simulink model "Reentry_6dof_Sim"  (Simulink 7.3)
settings: Solver=ode45  StartTime=0.0  StopTime=1943  FixedStep=0.01
InitFcn:
  | init
StopFcn:
  | pl
  | save_traj
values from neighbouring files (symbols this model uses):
  d2r = pi/180    (= 0.0174532925199)    [init.m]    (also in pl.m; robust.m)
  h0 = 250000.0    (= 250000)    [init.m]
  mass = 528.0    (= 528)    [init.m]
  r2d = 180/pi    (= 57.2957795131)    [init.m]    (also in pl.m; robust.m)
  sp = 15    [init.m]
  x0 = [0 0 -2 -2 0 0 18 0 0 0]'*d2r    [init.m]
  x_cg = -17.04    [init.m]
  x_ref = -16.2    [init.m]
  y_cg = 0    [init.m]
  z_cg = -2.03    [init.m]
  z_ref = -2.1    [init.m]
undefined symbols (not defined in the file or in its folder): Cl, Cld1, Cld2, Cld3, Cld4, Cld5, Cld6, Cld7, Cm, Cmd1, Cmd2, Cmd3, Cmd4, Cmd5, Cmd6, Cmd7, Cn, Cnd1, Cnd2, Cnd3, Cnd4, Cnd5, Cnd6, Cnd7, CX, CXd1, CXd2, CXd3, CXd4, CXd5, CXd6, CXd7, CY, CYd1, CYd2, CYd3, CYd4, CYd5, CYd6, CYd7, CZ, CZd1, CZd2, CZd3, CZd4, CZd5, CZd6, CZd7, ft, HDBK, km, Lateral_FCS, MIL, Pitch_FCS, sigbuilder_block
libraries: aerolibasang x3, aerolib6dof2 x1, aerolibconvert2 x1, aerolibatmos2 x1, aerolibgravity2 x1, aerolibadyn x1
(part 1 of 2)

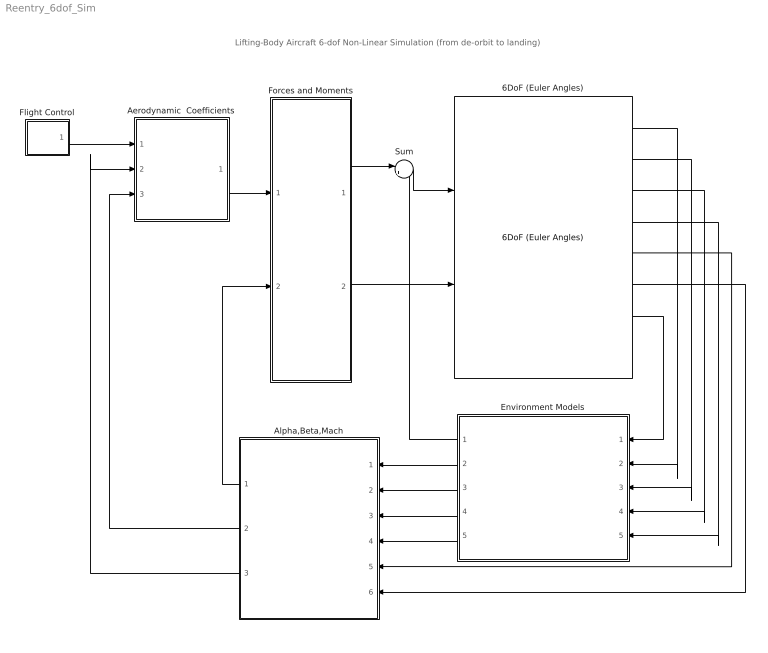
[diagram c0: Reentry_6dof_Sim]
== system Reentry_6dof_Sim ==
  note: Lifting-Body Aircraft 6-dof Non-Linear Simulation (from de-orbit to landing)
  6DoF (Euler Angles) : aerolib6dof2/6DoF (Euler Angles)  SystemSampleTime=-1  units=English (Velocity in ft/s)  mtype=Fixed  rep=Euler Angles  xme_0=[-x0, 0, -h0]  Vm_0=Uvw_0  eul_0=Euler_0  pm_0=pqr_0  mass_0=mass  mass_e=0.5  mass_f=2.0  inertia=inertia  inertia_e=eye(3)  inertia_f=2*eye(3)  k_quat=1.0
  Aerodynamic  Coefficients : Subsystem
  Alpha,Beta,Mach : Subsystem
  Environment Models : Subsystem
  Flight Control : Subsystem
  Forces and Moments : Subsystem
  Sum : Sum  Inputs=|++  OutDataType=sfix(16)  OutScaling=2^0
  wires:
  6DoF (Euler Angles)/5 -> Alpha,Beta,Mach/5(Vb)
  6DoF (Euler Angles)/1 -> Environment Models/2(Ve)
  6DoF (Euler Angles)/2 -> Environment Models/3(Xe)
  6DoF (Euler Angles)/3 -> Environment Models/4(Euler)
  6DoF (Euler Angles)/4 -> Environment Models/5(DCM)
  Sum/1 -> 6DoF (Euler Angles)/1
  Forces and Moments/1(X,Y,Z) -> Sum/1
  Environment Models/2(Speed of Sound) -> Alpha,Beta,Mach/1(Speed of Sound)
  Environment Models/3(Wind Velocity) -> Alpha,Beta,Mach/2(Wind Velocity)
  Environment Models/4(Air Density) -> Alpha,Beta,Mach/3(Air Density)
  Environment Models/5(Wind Angular Rates) -> Alpha,Beta,Mach/4(Wind Angular Rates)
  6DoF (Euler Angles)/6 -> Alpha,Beta,Mach/6(p,q,r)
  Forces and Moments/2(LMN) -> 6DoF (Euler Angles)/2
  6DoF (Euler Angles)/7 -> Environment Models/1(omgd)
  Environment Models/1(Fg) -> Sum/2
  Alpha,Beta,Mach/1(qbar) -> Forces and Moments/2(qbar)
  Aerodynamic  Coefficients/1(Coeff) -> Forces and Moments/1(Coeff)
  Alpha,Beta,Mach/2(Mach) -> Aerodynamic  Coefficients/3(Mach)
  Alpha,Beta,Mach/3(Incid) -> Aerodynamic  Coefficients/2(Incid)
  Flight Control/1(delta) -> Aerodynamic  Coefficients/1(deltas)

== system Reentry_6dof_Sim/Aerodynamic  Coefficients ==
  note: Aero Coefficients, funct. of: (Alpha, Beta, Mach#, Deflection)
  deltas : Inport  OutDataType=sfix(16)  OutScaling=2^0
  Incid : Inport  Port=2  OutDataType=sfix(16)  OutScaling=2^0
  Mach : Inport  Port=3  OutDataType=sfix(16)  OutScaling=2^0
  Aero-Surface Coefficient Increments : Subsystem
  Angle Conversion : aerolibconvert2/Angle Conversion  SystemSampleTime=-1  IU=rad  OU=deg
  Base Aero  Coefficients : Subsystem
  Sum : Sum  Inputs=|++  OutDataType=fixdt(1, 16)  OutScaling=2^0
  albet : Scope
  delta : Scope
  Coeff : Outport  OutDataType=sfix(16)  OutScaling=2^0  InitialOutput=0
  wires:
  deltas/1 -> Aero-Surface Coefficient Increments/3(delta), delta/1
  Base Aero  Coefficients/1(Coeff) -> Sum/1
  Sum/1 -> Coeff/1
  Mach/1 -> Base Aero  Coefficients/2(Mach), Aero-Surface Coefficient Increments/2(Mach)
  Angle Conversion/1 -> Base Aero  Coefficients/1(albet), albet/1, Aero-Surface Coefficient Increments/1(albet)
  Incid/1 -> Angle Conversion/1
  Aero-Surface Coefficient Increments/1(Coeff) -> Sum/2

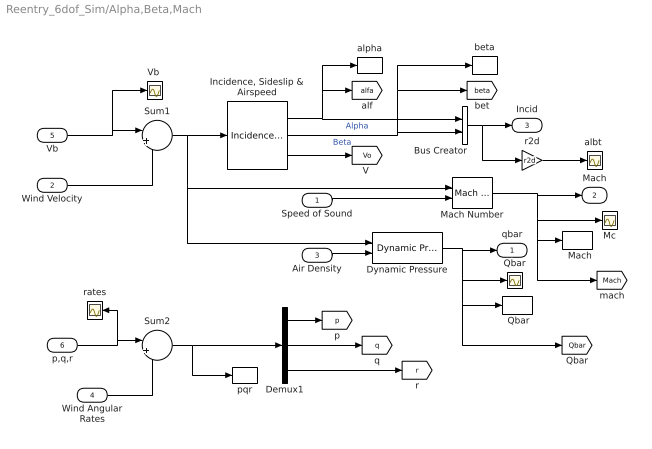
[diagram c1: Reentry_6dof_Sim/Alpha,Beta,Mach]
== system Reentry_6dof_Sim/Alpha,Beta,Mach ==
  Speed of Sound : Inport  OutDataType=sfix(16)  OutScaling=2^0
  Wind Velocity : Inport  Port=2  PortDimensions=3  OutDataType=sfix(16)  OutScaling=2^0
  Air Density : Inport  Port=3  OutDataType=sfix(16)  OutScaling=2^0
  Wind Angular Rates : Inport  Port=4  PortDimensions=3  OutDataType=sfix(16)  OutScaling=2^0
  Vb : Inport  Port=5  PortDimensions=3  OutDataType=sfix(16)  OutScaling=2^0
  p,q,r : Inport  Port=6  PortDimensions=3  OutDataType=sfix(16)  OutScaling=2^0
  "  Mach" : ToWorkspace  VariableName=Mach  SampleTime=-1  SaveFormat=Array
  " Qbar" : ToWorkspace  VariableName=Qbar  SampleTime=-1  SaveFormat=Array
  Bus Creator : BusCreator  Inputs=2
  Demux1 : Demux  Outputs=3
  Dynamic Pressure : aerolibasang/Dynamic Pressure  SystemSampleTime=-1
  "Incidence, Sideslip & Airspeed" : aerolibasang/Incidence, Sideslip, & Airspeed  SystemSampleTime=-1
  Mach Number : aerolibasang/Mach Number  SystemSampleTime=-1
  Mc : Scope
  Qbar : Scope
  Sum1 : Sum  Inputs=|+-  OutDataType=sfix(16)  OutScaling=2^0
  Sum2 : Sum  Inputs=|++  OutDataType=sfix(16)  OutScaling=2^0
  "Vb " : Scope
  "albt " : Scope
  alpha : ToWorkspace  VariableName=alfa  SampleTime=-1  SaveFormat=Array
  beta : ToWorkspace  VariableName=beta  SampleTime=-1  SaveFormat=Array
  pqr : ToWorkspace  VariableName=pqr  SampleTime=-1  SaveFormat=Array
  r2d : Gain  Gain=r2d  ParameterDataType=sfix(16)  ParameterScaling=2^0  OutDataType=sfix(16)  OutScaling=2^0
  rates : Scope
  qbar : Outport  OutDataType=sfix(16)  OutScaling=2^0  InitialOutput=0
  Mach : Outport  Port=2  OutDataType=sfix(16)  OutScaling=2^0
  Incid : Outport  Port=3  OutDataType=sfix(16)  OutScaling=2^0
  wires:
  Demux1/1 -> [p]
  Demux1/3 -> [r]
  Demux1/2 -> [q]
  Sum2/1 -> pqr/1, Demux1/1
  Wind Angular Rates/1 -> Sum2/2
  p,q,r/1 -> rates/1, Sum2/1
  "Incidence, Sideslip & Airspeed"/1 -> alpha/1, [alfa], Bus Creator/1  "Alpha"
  Bus Creator/1 -> Incid/1, r2d/1
  "Incidence, Sideslip & Airspeed"/2 -> beta/1, [beta], Bus Creator/2  "Beta"
  Wind Velocity/1 -> Sum1/2
  Speed of Sound/1 -> Mach Number/2
  Vb/1 -> "Vb "/1, Sum1/1
  Sum1/1 -> "Incidence, Sideslip & Airspeed"/1, Mach Number/1, Dynamic Pressure/1
  Mach Number/1 -> [Mach], "  Mach"/1, Mc/1, Mach/1
  Air Density/1 -> Dynamic Pressure/2
  Dynamic Pressure/1 -> [Qbar], " Qbar"/1, Qbar/1, qbar/1
  "Incidence, Sideslip & Airspeed"/3 -> [Vo]
  r2d/1 -> "albt "/1

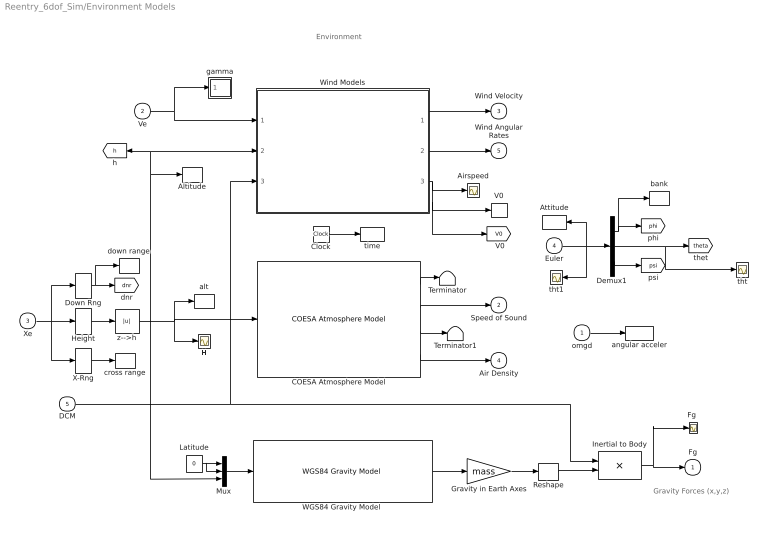
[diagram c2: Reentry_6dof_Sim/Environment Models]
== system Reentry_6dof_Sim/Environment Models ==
  note: Gravity Forces (x,y,z)
  note: Environment
  omgd : Inport  OutDataType=sfix(16)  OutScaling=2^0
  Ve : Inport  Port=2  OutDataType=sfix(16)  OutScaling=2^0
  Xe : Inport  Port=3  PortDimensions=3  OutDataType=sfix(16)  OutScaling=2^0
  Euler : Inport  Port=4  OutDataType=sfix(16)  OutScaling=2^0
  DCM : Inport  Port=5  OutDataType=sfix(16)  OutScaling=2^0
  Airspeed : Scope
  Altitude : ToWorkspace  VariableName=Alt  SampleTime=-1  SaveFormat=Array
  Attitude : ToWorkspace  VariableName=Euler  SampleTime=-1  SaveFormat=Array
  COESA Atmosphere Model : aerolibatmos2/COESA Atmosphere Model  SystemSampleTime=-1  units=English (Velocity in ft/s)  spec=MIL-HDBK-310  model=Profile  profile_var=High temperature  profile_percent=1%  profile_alt=40 km (131234 ft)  envelope_var=High temperature  envelope_percent=1%  action=Warning
  Clock : Clock
  Demux1 : Demux  Outputs=3
  Down Rng : Selector  InputPortWidth=3  IndexOptions=Index vector (dialog)  Indices=[1]  OutputSizes=1
  "Fg " : Scope
  Gravity in Earth Axes : Gain  Gain=mass  ParameterDataType=sfix(16)  ParameterScaling=2^0  OutDataType=sfix(16)  OutScaling=2^0
  H : Scope
  Height : Selector  InputPortWidth=3  IndexOptions=Index vector (dialog)  Indices=[3]  OutputSizes=1
  Inertial to Body : Product  Multiplication=Matrix(*)  OutDataType=sfix(16)  OutScaling=2^0
  Latitude : Constant  Value=0  OutDataType=sfix(16)  OutScaling=2^0
  Mux : Mux  Inputs=3
  Reshape : Reshape
  Terminator : Terminator
  Terminator1 : Terminator
  V0 : ToWorkspace  VariableName=V0  SampleTime=-1  SaveFormat=Array
  "WGS84 Gravity Model " : aerolibgravity2/WGS84 Gravity Model   SystemSampleTime=-1  model=WGS84 Taylor Series  units=English  no_atmos=on  precessing=on  jd_loc=off  month=October  day=10  year=2004  no_centrifugal=on  action=None
  Wind Models : Subsystem
  X-Rng : Selector  InputPortWidth=3  IndexOptions=Index vector (dialog)  Indices=[2]  OutputSizes=1
  alt : ToWorkspace  VariableName=alt  SampleTime=-1  SaveFormat=Array
  angular acceler : ToWorkspace  VariableName=omgd  SampleTime=-1  SaveFormat=Array
  bank : ToWorkspace  VariableName=phi  SampleTime=-1  SaveFormat=Array
  cross range : ToWorkspace  VariableName=xrng  SampleTime=-1  SaveFormat=Array
  down range : ToWorkspace  VariableName=dnr  SampleTime=-1  SaveFormat=Array
  gamma : Subsystem
  tht : Scope
  tht1 : Scope
  time : ToWorkspace  VariableName=time  SampleTime=-1  SaveFormat=Array
  z-->h : Abs
  Fg : Outport  OutDataType=sfix(16)  OutScaling=2^0  InitialOutput=0
  Speed of Sound : Outport  Port=2  OutDataType=sfix(16)  OutScaling=2^0  InitialOutput=0
  Wind Velocity : Outport  Port=3  OutDataType=sfix(16)  OutScaling=2^0  InitialOutput=0
  Air Density : Outport  Port=4  OutDataType=sfix(16)  OutScaling=2^0  InitialOutput=0
  Wind Angular Rates : Outport  Port=5  OutDataType=sfix(16)  OutScaling=2^0  InitialOutput=0
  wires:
  Reshape/1 -> Inertial to Body/2
  "WGS84 Gravity Model "/1 -> Gravity in Earth Axes/1
  Gravity in Earth Axes/1 -> Reshape/1
  COESA Atmosphere Model/1 -> Terminator/1
  COESA Atmosphere Model/2 -> Speed of Sound/1
  COESA Atmosphere Model/3 -> Terminator1/1
  COESA Atmosphere Model/4 -> Air Density/1
  DCM/1 -> Inertial to Body/1, Wind Models/3(DCM)
  Inertial to Body/1 -> Fg/1, "Fg "/1
  Mux/1 -> "WGS84 Gravity Model "/1
  Latitude/1 -> Mux/2, Mux/1
  Height/1 -> z-->h/1
  Xe/1 -> Height/1, Down Rng/1, X-Rng/1
  z-->h/1 -> COESA Atmosphere Model/1, H/1, alt/1, Mux/3, Wind Models/2(Altitude), [h], Altitude/1
  Wind Models/2(pg,qg,rg) -> Wind Angular Rates/1
  Wind Models/3(Airspeed) -> Airspeed/1, V0/1, [V0]
  Ve/1 -> Wind Models/1(Ve), gamma/1(Ve)
  Wind Models/1(ug,vg,wg) -> Wind Velocity/1
  Down Rng/1 -> [dnr], down range/1
  Clock/1 -> time/1
  X-Rng/1 -> cross range/1
  omgd/1 -> angular acceler/1
  Euler/1 -> Demux1/1, Attitude/1, tht1/1
  Demux1/2 -> [theta], tht/1
  Demux1/1 -> [phi], bank/1
  Demux1/3 -> [psi]

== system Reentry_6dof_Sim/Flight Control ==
  note: Surface Open-Loop Trim Commands and Closed-Loop Flight Control
  Bus Creator2 : BusCreator  Inputs=7
  Deflection Limits : Subsystem
  Demux1 : Demux  Outputs=7
  Flight  Control : Subsystem
  Sum1 : Sum  Inputs=|++  OutDataType=fixdt(1, 16)  OutScaling=2^0
  Trim Cmds : Subsystem
  delta : Outport
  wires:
  Trim Cmds/1(Trim) -> Sum1/2
  Flight  Control/1(deltas) -> Sum1/1
  Sum1/1 -> Deflection Limits/1(In)
  Demux1/1 -> Bus Creator2/1  "Left_Elevon"
  Bus Creator2/1 -> delta/1
  Demux1/2 -> Bus Creator2/2  "Right_Elevon"
  Demux1/3 -> Bus Creator2/3  "Vert_Rudder"
  Demux1/6 -> Bus Creator2/6  "Bflap_LoLft"
  Demux1/7 -> Bus Creator2/7  "Bflap_LoRht"
  Demux1/5 -> Bus Creator2/5  "Bflap_UpRht"
  Demux1/4 -> Bus Creator2/4  "Bflap_UpLft"
  Deflection Limits/1(Ou) -> Demux1/1

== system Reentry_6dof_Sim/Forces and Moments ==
  note: Aero coefficients (CX,CY,CZ,Cl,Cm,Cn)
  note: Dynamic Pressure
  note: Moments and Forces due to Aero and Engine Thrust
  Coeff : Inport  OutDataType=sfix(16)  OutScaling=2^0
  qbar : Inport  Port=2  OutDataType=sfix(16)  OutScaling=2^0
  Acceler X,Y,Z : Scope
  Aero-Forcces : Selector  InputPortWidth=3  IndexOptions=Index vector (dialog)  Indices=[3,1,2]  OutputSizes=1
  "Aerodynamic Forces and Moments (Fx,Fy,Fz), (Lx,My,Nz)" : aerolibadyn/Aerodynamic Forces and Moments   SystemSampleTime=-1  inputAxes=Body  outputForceAxes=Body  outputMomentAxes=Body  S=Sref  b=sp  cbar=ch
  Axyz : ToWorkspace  VariableName=Axyz  SampleTime=-1  SaveFormat=Array
  "Center of Gravity plus Variation [x_cg, y_cg,  z_cg]" : Step  Time=0  Before="[x_cg, y_cg,  z_cg]"  After="[x_cg,   y_cg,   z_cg]"
  Faero : ToWorkspace  VariableName=Flds  SampleTime=-1  SaveFormat=Array
  "Force " : Scope
  Force ---> Acc : Gain  Gain=1/mass  ParameterDataType=sfix(16)  ParameterScaling=2^0  OutDataType=sfix(16)  OutScaling=2^0
  Moments : Scope
  Moments Reference Center (MRC) in (feet) : Constant  Value=[x_ref 0 z_ref]  OutDataType=sfix(16)  OutScaling=2^0
  Nz : Selector  InputPortWidth=3  IndexOptions=Index vector (dialog)  Indices=[3]  OutputSizes=1
  X,Y,Z : Outport  OutDataType=sfix(16)  OutScaling=2^0  InitialOutput=0
  LMN : Outport  Port=2  OutDataType=sfix(16)  OutScaling=2^0  InitialOutput=0
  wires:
  Coeff/1 -> "Aerodynamic Forces and Moments (Fx,Fy,Fz), (Lx,My,Nz)"/1
  qbar/1 -> "Aerodynamic Forces and Moments (Fx,Fy,Fz), (Lx,My,Nz)"/2
  Moments Reference Center (MRC) in (feet)/1 -> "Aerodynamic Forces and Moments (Fx,Fy,Fz), (Lx,My,Nz)"/4
  "Center of Gravity plus Variation [x_cg, y_cg,  z_cg]"/1 -> "Aerodynamic Forces and Moments (Fx,Fy,Fz), (Lx,My,Nz)"/3
  Force ---> Acc/1 -> Acceler X,Y,Z/1, Axyz/1, Nz/1
  Aero-Forcces/1 -> Faero/1
  "Aerodynamic Forces and Moments (Fx,Fy,Fz), (Lx,My,Nz)"/2 -> LMN/1, Moments/1
  "Aerodynamic Forces and Moments (Fx,Fy,Fz), (Lx,My,Nz)"/1 -> Aero-Forcces/1, Force ---> Acc/1, X,Y,Z/1, "Force "/1
  Nz/1 -> [Nz]

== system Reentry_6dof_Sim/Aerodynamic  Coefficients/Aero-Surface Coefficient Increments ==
  note: Surface Coefficients
  albet : Inport
  Mach : Inport  Port=2
  delta : Inport  Port=3
  LL Bflap : Subsystem
  LR Bflap : Subsystem
  Left Elevon : Subsystem
  Right Elevon : Subsystem
  Rudder : Subsystem
  Sum : Sum  Inputs=+++++++  OutDataType=fixdt(1, 16)  OutScaling=2^0
  UL Bflap : Subsystem
  UR Bflap : Subsystem
  Coeff : Outport
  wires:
  Left Elevon/1(Coeff) -> Sum/1
  delta/1 -> Left Elevon/3(delta), Right Elevon/3(delta), Rudder/3(delta), UL Bflap/3(delta), UR Bflap/3(delta), LL Bflap/3(delta), LR Bflap/3(delta)
  albet/1 -> Left Elevon/1(albet), Right Elevon/1(albet), Rudder/1(albet), UL Bflap/1(albet), UR Bflap/1(albet), LL Bflap/1(albet), LR Bflap/1(albet)
  Mach/1 -> Left Elevon/2(Mach), Right Elevon/2(Mach), Rudder/2(Mach), UL Bflap/2(Mach), UR Bflap/2(Mach), LL Bflap/2(Mach), LR Bflap/2(Mach)
  Sum/1 -> Coeff/1
  Right Elevon/1(Coeff) -> Sum/2
  Rudder/1(Coeff) -> Sum/3
  UL Bflap/1(Coeff) -> Sum/4
  UR Bflap/1(Coeff) -> Sum/5
  LL Bflap/1(Coeff) -> Sum/6
  LR Bflap/1(Coeff) -> Sum/7

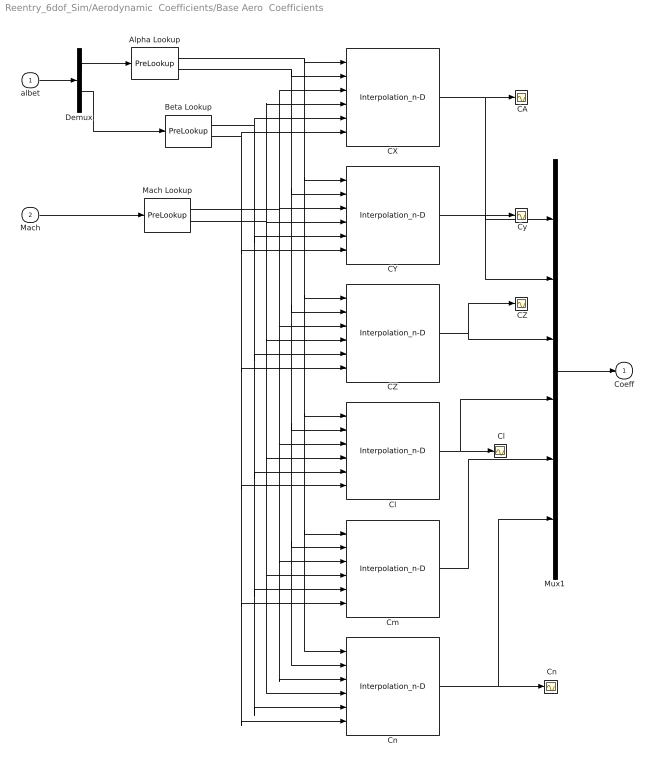
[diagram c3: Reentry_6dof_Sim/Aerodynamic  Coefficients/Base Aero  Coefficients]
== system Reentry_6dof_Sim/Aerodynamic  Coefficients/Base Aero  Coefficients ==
  albet : Inport  OutDataType=sfix(16)  OutScaling=2^0
  Mach : Inport  Port=2  OutDataType=sfix(16)  OutScaling=2^0
  " CA" : Scope
  " CZ" : Scope
  " Cl" : Scope
  " Cn" : Scope
  " Cy" : Scope
  Alpha Lookup : PreLookup  BreakpointsData=Alfas  BeginIndexSearchUsingPreviousIndexResult=on  ProcessOutOfRangeInput=Linear extrapolation  IndexDataType=sfix(16)  FractionDataType=sfix(16)  FractionScaling=2^0
  Beta Lookup : PreLookup  BreakpointsData=Betas  BeginIndexSearchUsingPreviousIndexResult=on  ProcessOutOfRangeInput=Linear extrapolation  IndexDataType=sfix(16)  FractionDataType=sfix(16)  FractionScaling=2^0
  CX : Interpolation_n-D  NumberOfTableDimensions=3  Table=CX  CheckIndexInCode=off  OutDataType=sfix(16)  OutScaling=2^0
  CY : Interpolation_n-D  NumberOfTableDimensions=3  Table=CY  CheckIndexInCode=off  OutDataType=sfix(16)  OutScaling=2^0
  CZ : Interpolation_n-D  NumberOfTableDimensions=3  Table=CZ  CheckIndexInCode=off  OutDataType=sfix(16)  OutScaling=2^0
  Cl : Interpolation_n-D  NumberOfTableDimensions=3  Table=Cl  CheckIndexInCode=off  OutDataTypeMode=double  OutDataType=sfix(16)  OutScaling=2^0  OutDataTypeStr=double
  Cm : Interpolation_n-D  NumberOfTableDimensions=3  Table=Cm  CheckIndexInCode=off  OutDataType=sfix(16)  OutScaling=2^0
  Cn : Interpolation_n-D  NumberOfTableDimensions=3  Table=Cn  CheckIndexInCode=off  OutDataType=sfix(16)  OutScaling=2^0
  Demux : Demux  Outputs=2
  Mach Lookup : PreLookup  BreakpointsData=Machs  BeginIndexSearchUsingPreviousIndexResult=on  ProcessOutOfRangeInput=Linear extrapolation  IndexDataType=sfix(16)  FractionDataType=sfix(16)  FractionScaling=2^0
  Mux1 : Mux  Inputs=6
  Coeff : Outport  OutDataType=sfix(16)  OutScaling=2^0  InitialOutput=0
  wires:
  Mach/1 -> Mach Lookup/1
  albet/1 -> Demux/1
  Demux/2 -> Beta Lookup/1
  Mux1/1 -> Coeff/1
  Beta Lookup/2 -> CZ/6, Cl/6, Cn/6, Cm/6, CY/6, CX/6
  Beta Lookup/1 -> CY/5, CZ/5, Cl/5, Cn/5, Cm/5, CX/5
  Mach Lookup/2 -> CX/4, CZ/4, Cl/4, Cn/4, Cm/4, CY/4
  Mach Lookup/1 -> CX/3, CZ/3, Cl/3, Cn/3, Cm/3, CY/3
  Alpha Lookup/2 -> Cn/2, Cm/2, Cl/2, CZ/2, CY/2, CX/2
  Alpha Lookup/1 -> CZ/1, Cl/1, Cn/1, Cm/1, CY/1, CX/1
  Cn/1 -> " Cn"/1, Mux1/6
  Cm/1 -> Mux1/5
  Cl/1 -> " Cl"/1, Mux1/4
  CZ/1 -> " CZ"/1, Mux1/3
  CY/1 -> " Cy"/1, Mux1/2
  CX/1 -> " CA"/1, Mux1/1
  Demux/1 -> Alpha Lookup/1

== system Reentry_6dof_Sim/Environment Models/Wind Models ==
  note: Wind Disturbance Model (Shear, Gust, Turbulence)
  Ve : Inport  OutDataType=sfix(16)  OutScaling=2^0
  Altitude : Inport  Port=2  OutDataType=sfix(16)  OutScaling=2^0
  DCM : Inport  Port=3  OutDataType=sfix(16)  OutScaling=2^0
  Dot Product : DotProduct  OutDataType=sfix(16)  OutScaling=2^-10  SaturateOnIntegerOverflow=on
  V : Math  Operator=sqrt  OutDataType=sfix(16)  OutScaling=2^0
  ug,vg,wg : Outport  OutDataType=sfix(16)  OutScaling=2^0
  pg,qg,rg : Outport  Port=2  OutDataType=sfix(16)  OutScaling=2^0
  Airspeed : Outport  Port=3  OutDataType=sfix(16)  OutScaling=2^0
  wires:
  Altitude/1 -> ?
  Dot Product/1 -> V/1
  Ve/1 -> Dot Product/1, Dot Product/2
  V/1 -> Airspeed/1

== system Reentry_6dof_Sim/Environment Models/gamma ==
  Ve : Inport
  -1 : Gain  Gain=-1  ParameterDataType=sfix(16)  ParameterScaling=2^0  OutDataType=sfix(16)  OutScaling=2^0
  57.2 : Gain  Gain=r2d  ParameterDataType=sfix(16)  ParameterScaling=2^0  OutDataType=sfix(16)  OutScaling=2^0
  Vx : Selector  InputPortWidth=3  IndexOptions=Index vector (dialog)  Indices=[1]  OutputSizes=1
  Vz : Selector  InputPortWidth=3  IndexOptions=Index vector (dialog)  Indices=[3]  OutputSizes=1
  atan : Trigonometry  Operator=atan2
  "gam " : Scope
  gama : ToWorkspace  VariableName=gama  SampleTime=-1  SaveFormat=Array
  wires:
  Vz/1 -> atan/1
  Vx/1 -> atan/2
  atan/1 -> 57.2/1
  57.2/1 -> "gam "/1, gama/1, [gama]
  -1/1 -> Vz/1
  Ve/1 -> -1/1, Vx/1

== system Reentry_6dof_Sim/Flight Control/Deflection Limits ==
  In : Inport
  "  Delta  (deg)" : ToWorkspace  VariableName=delta  SampleTime=-1  SaveFormat=Array
  Demux : Demux  Outputs=7
  LL BFlap : Saturate  UpperLimit=60  LowerLimit=0  OutDataType=fixdt(1, 16)  OutScaling=2^0
  LR BFlap : Saturate  UpperLimit=60  LowerLimit=0  OutDataType=fixdt(1, 16)  OutScaling=2^0
  Left Elev : Saturate  UpperLimit=30  LowerLimit=-30  OutDataType=fixdt(1, 16)  OutScaling=2^0
  Mux1 : Mux  Inputs=7
  Right Elev : Saturate  UpperLimit=30  LowerLimit=-30  OutDataType=fixdt(1, 16)  OutScaling=2^0
  UL BFlap : Saturate  UpperLimit=0  LowerLimit=-60  OutDataType=fixdt(1, 16)  OutScaling=2^0
  UR BFlap : Saturate  UpperLimit=0  LowerLimit=-60  OutDataType=fixdt(1, 16)  OutScaling=2^0
  Vert Rudder : Saturate  UpperLimit=40  LowerLimit=-40  OutDataType=fixdt(1, 16)  OutScaling=2^0
  Ou : Outport
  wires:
  Mux1/1 -> Ou/1, "  Delta  (deg)"/1
  In/1 -> Demux/1
  Demux/7 -> LR BFlap/1
  Demux/6 -> LL BFlap/1
  Demux/5 -> UR BFlap/1
  Demux/4 -> UL BFlap/1
  Demux/3 -> Vert Rudder/1
  Demux/2 -> Right Elev/1
  Demux/1 -> Left Elev/1
  LL BFlap/1 -> Mux1/6
  UR BFlap/1 -> Mux1/5
  UL BFlap/1 -> Mux1/4
  Vert Rudder/1 -> Mux1/3
  Right Elev/1 -> Mux1/2
  Left Elev/1 -> Mux1/1
  LR BFlap/1 -> Mux1/7

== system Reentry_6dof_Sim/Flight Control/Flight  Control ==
  note: Guidance Commands and Flight Control System
  note: 7 Aero-Surface Deflections
  Guidance Commands 1876 sec : Subsystem  Tag=STV Subsys  LoadFcn=sigbuilder_block('load');  StartFcn=sigbuilder_block('start');  StopFcn=sigbuilder_block('stop');  ClipboardFcn=sigbuilder_block('clipboard');
  Lateral Flight Control : Subsystem
  Pitch Flight Control : Subsystem
  Sum : Sum  Inputs=|+-  OutDataType=fixdt(1, 16)  OutScaling=2^0
  Sum1 : Sum  Inputs=|-+  OutDataType=fixdt(1, 16)  OutScaling=2^0
  Sum4 : Sum  Inputs=|++  OutDataType=fixdt(1, 16)  OutScaling=2^0
  d2r : Gain  Gain=d2r  ParameterDataType=fixdt(1, 16)  ParameterScaling=2^0  OutDataType=fixdt(1, 16)  OutScaling=2^0
  deltas : Outport
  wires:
  Guidance Commands 1876 sec/1(Alpha_cmd) -> d2r/1
  Pitch Flight Control/1(delta) -> Sum4/1
  Sum4/1 -> deltas/1
  Lateral Flight Control/1(delta) -> Sum4/2
  [alfa] -> Sum/1
  Sum/1 -> Pitch Flight Control/2(alfer), Lateral Flight Control/1(alfe)  "alfer"
  Guidance Commands 1876 sec/2(Gamma_cmd) -> Sum1/1
  [gama] -> Sum1/2
  Sum1/1 -> Pitch Flight Control/1(gamer)
  d2r/1 -> Sum/2

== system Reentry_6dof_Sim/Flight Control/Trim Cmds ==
  Body-Flap Trims : Subsystem  Tag=STV Subsys  LoadFcn=sigbuilder_block('load');  StartFcn=sigbuilder_block('start');  StopFcn=sigbuilder_block('stop');  ClipboardFcn=sigbuilder_block('clipboard');
  Elevon Trims : Subsystem  Tag=STV Subsys  LoadFcn=sigbuilder_block('load');  StartFcn=sigbuilder_block('start');  StopFcn=sigbuilder_block('stop');  ClipboardFcn=sigbuilder_block('clipboard');
  Mux3 : Mux  Inputs=7
  rudder : Constant  Value=0  OutDataType=fixdt(1, 16)  OutScaling=2^0
  Trim : Outport
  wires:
  Elevon Trims/1(Left Elev) -> Mux3/1
  Elevon Trims/2(Right Elev) -> Mux3/2
  rudder/1 -> Mux3/3
  Body-Flap Trims/1(Up-Left BF) -> Mux3/4
  Body-Flap Trims/2(Up Right BF) -> Mux3/5
  Body-Flap Trims/3(Lo-Left BF) -> Mux3/6
  Body-Flap Trims/4(Lo-Right BF) -> Mux3/7
  Mux3/1 -> Trim/1

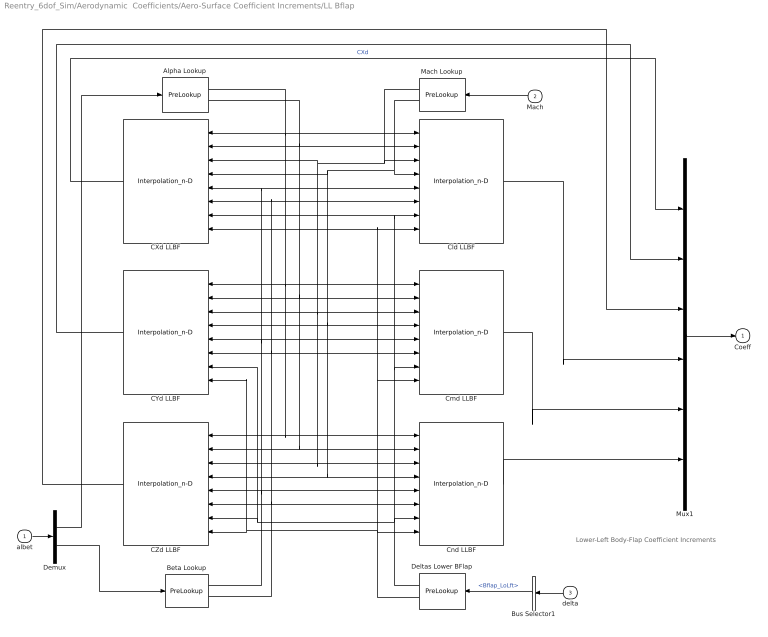
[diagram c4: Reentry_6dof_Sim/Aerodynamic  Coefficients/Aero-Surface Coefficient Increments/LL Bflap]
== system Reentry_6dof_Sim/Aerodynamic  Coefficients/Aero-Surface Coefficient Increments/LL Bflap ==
  note: Lower-Left Body-Flap Coefficient Increments
  albet : Inport  OutDataType=sfix(16)  OutScaling=2^0
  Mach : Inport  Port=2  OutDataType=sfix(16)  OutScaling=2^0
  delta : Inport  Port=3  OutDataType=sfix(16)  OutScaling=2^0
  Alpha Lookup : PreLookup  BreakpointsData=Alfas  BeginIndexSearchUsingPreviousIndexResult=on  ProcessOutOfRangeInput=Linear extrapolation  IndexDataType=sfix(16)  FractionDataType=sfix(16)  FractionScaling=2^0
  Beta Lookup : PreLookup  BreakpointsData=Betas  BeginIndexSearchUsingPreviousIndexResult=on  ProcessOutOfRangeInput=Linear extrapolation  IndexDataType=sfix(16)  FractionDataType=sfix(16)  FractionScaling=2^0
  Bus Selector1 : BusSelector  OutputSignals=Bflap_LoLft
  CXd LLBF : Interpolation_n-D  NumberOfTableDimensions=4  Table=CXd6  CheckIndexInCode=off  OutDataType=sfix(16)  OutScaling=2^0
  CYd LLBF : Interpolation_n-D  NumberOfTableDimensions=4  Table=CYd6  CheckIndexInCode=off  OutDataType=sfix(16)  OutScaling=2^0
  CZd LLBF : Interpolation_n-D  NumberOfTableDimensions=4  Table=CZd6  CheckIndexInCode=off  OutDataType=sfix(16)  OutScaling=2^0
  Cld LLBF : Interpolation_n-D  NumberOfTableDimensions=4  Table=Cld6  CheckIndexInCode=off  OutDataType=sfix(16)  OutScaling=2^0
  Cmd LLBF : Interpolation_n-D  NumberOfTableDimensions=4  Table=Cmd6  CheckIndexInCode=off  OutDataType=sfix(16)  OutScaling=2^0
  Cnd LLBF : Interpolation_n-D  NumberOfTableDimensions=4  Table=Cnd6  CheckIndexInCode=off  OutDataType=sfix(16)  OutScaling=2^0
  Deltas Lower BFlap : PreLookup  BreakpointsData=Deltas6  BeginIndexSearchUsingPreviousIndexResult=on  ProcessOutOfRangeInput=Linear extrapolation  IndexDataType=sfix(16)  FractionDataType=sfix(16)  FractionScaling=2^0
  Demux : Demux  Outputs=2
  Mach Lookup : PreLookup  BreakpointsData=Machs  BeginIndexSearchUsingPreviousIndexResult=on  ProcessOutOfRangeInput=Linear extrapolation  IndexDataType=sfix(16)  FractionDataType=sfix(16)  FractionScaling=2^0
  Mux1 : Mux  Inputs=6
  Coeff : Outport  OutDataType=sfix(16)  OutScaling=2^0  InitialOutput=0
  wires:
  CZd LLBF/1 -> Mux1/3
  CYd LLBF/1 -> Mux1/2
  CXd LLBF/1 -> Mux1/1  "CXd"
  Demux/2 -> Beta Lookup/1
  Mach/1 -> Mach Lookup/1
  Demux/1 -> Alpha Lookup/1
  Cld LLBF/1 -> Mux1/4
  Cmd LLBF/1 -> Mux1/5
  Cnd LLBF/1 -> Mux1/6
  Mux1/1 -> Coeff/1
  Deltas Lower BFlap/2 -> CXd LLBF/8, Cld LLBF/8, Cmd LLBF/8, Cnd LLBF/8, CYd LLBF/8, CZd LLBF/8
  Deltas Lower BFlap/1 -> CXd LLBF/7, Cld LLBF/7, Cmd LLBF/7, Cnd LLBF/7, CYd LLBF/7, CZd LLBF/7
  Beta Lookup/2 -> Cld LLBF/6, CXd LLBF/6, Cmd LLBF/6, CYd LLBF/6, Cnd LLBF/6, CZd LLBF/6
  Beta Lookup/1 -> Cld LLBF/5, CXd LLBF/5, Cmd LLBF/5, CYd LLBF/5, Cnd LLBF/5, CZd LLBF/5
  Mach Lookup/2 -> Cnd LLBF/4, CZd LLBF/4, Cmd LLBF/4, CYd LLBF/4, CXd LLBF/4, Cld LLBF/4
  Mach Lookup/1 -> Cnd LLBF/3, CZd LLBF/3, Cmd LLBF/3, CYd LLBF/3, CXd LLBF/3, Cld LLBF/3
  Alpha Lookup/2 -> Cnd LLBF/2, CZd LLBF/2, Cmd LLBF/2, CYd LLBF/2, Cld LLBF/2, CXd LLBF/2
  Alpha Lookup/1 -> Cnd LLBF/1, CZd LLBF/1, Cmd LLBF/1, CYd LLBF/1, Cld LLBF/1, CXd LLBF/1
  albet/1 -> Demux/1
  Bus Selector1/1 -> Deltas Lower BFlap/1  "<Bflap_LoLft>"
  delta/1 -> Bus Selector1/1

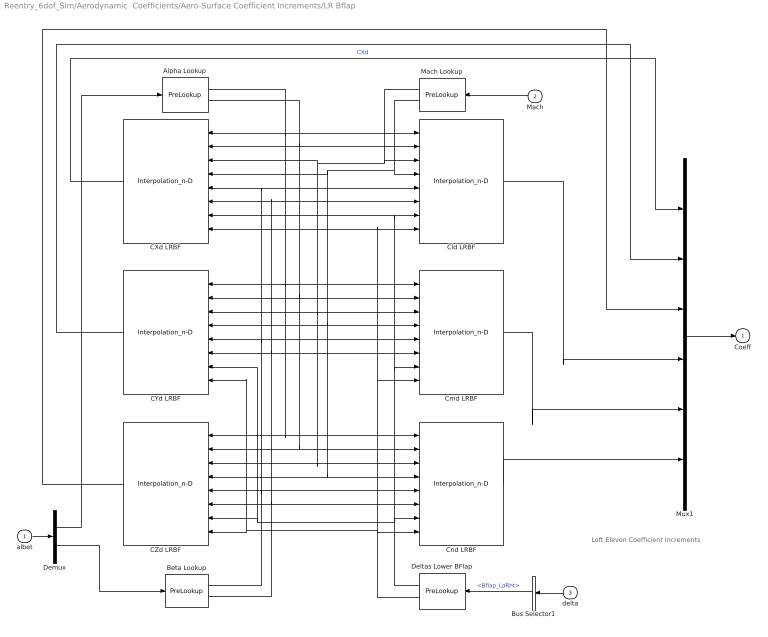
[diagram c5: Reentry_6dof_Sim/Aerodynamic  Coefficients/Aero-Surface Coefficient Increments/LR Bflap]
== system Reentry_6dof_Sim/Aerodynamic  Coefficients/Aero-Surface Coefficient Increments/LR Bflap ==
  note: Left Elevon Coefficient Increments
  albet : Inport  OutDataType=sfix(16)  OutScaling=2^0
  Mach : Inport  Port=2  OutDataType=sfix(16)  OutScaling=2^0
  delta : Inport  Port=3  OutDataType=sfix(16)  OutScaling=2^0
  Alpha Lookup : PreLookup  BreakpointsData=Alfas  BeginIndexSearchUsingPreviousIndexResult=on  ProcessOutOfRangeInput=Linear extrapolation  IndexDataType=sfix(16)  FractionDataType=sfix(16)  FractionScaling=2^0
  Beta Lookup : PreLookup  BreakpointsData=Betas  BeginIndexSearchUsingPreviousIndexResult=on  ProcessOutOfRangeInput=Linear extrapolation  IndexDataType=sfix(16)  FractionDataType=sfix(16)  FractionScaling=2^0
  Bus Selector1 : BusSelector  OutputSignals=Bflap_LoRht
  CXd LRBF : Interpolation_n-D  NumberOfTableDimensions=4  Table=CXd7  CheckIndexInCode=off  OutDataType=sfix(16)  OutScaling=2^0
  CYd LRBF : Interpolation_n-D  NumberOfTableDimensions=4  Table=CYd7  CheckIndexInCode=off  OutDataType=sfix(16)  OutScaling=2^0
  CZd LRBF : Interpolation_n-D  NumberOfTableDimensions=4  Table=CZd7  CheckIndexInCode=off  OutDataType=sfix(16)  OutScaling=2^0
  Cld LRBF : Interpolation_n-D  NumberOfTableDimensions=4  Table=Cld7  CheckIndexInCode=off  OutDataType=sfix(16)  OutScaling=2^0
  Cmd LRBF : Interpolation_n-D  NumberOfTableDimensions=4  Table=Cmd7  CheckIndexInCode=off  OutDataType=sfix(16)  OutScaling=2^0
  Cnd LRBF : Interpolation_n-D  NumberOfTableDimensions=4  Table=Cnd7  CheckIndexInCode=off  OutDataType=sfix(16)  OutScaling=2^0
  Deltas Lower BFlap : PreLookup  BreakpointsData=Deltas7  BeginIndexSearchUsingPreviousIndexResult=on  ProcessOutOfRangeInput=Linear extrapolation  IndexDataType=sfix(16)  FractionDataType=sfix(16)  FractionScaling=2^0
  Demux : Demux  Outputs=2
  Mach Lookup : PreLookup  BreakpointsData=Machs  BeginIndexSearchUsingPreviousIndexResult=on  ProcessOutOfRangeInput=Linear extrapolation  IndexDataType=sfix(16)  FractionDataType=sfix(16)  FractionScaling=2^0
  Mux1 : Mux  Inputs=6
  Coeff : Outport  OutDataType=sfix(16)  OutScaling=2^0  InitialOutput=0
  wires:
  CZd LRBF/1 -> Mux1/3
  CYd LRBF/1 -> Mux1/2
  CXd LRBF/1 -> Mux1/1  "CXd"
  Demux/2 -> Beta Lookup/1
  Mach/1 -> Mach Lookup/1
  Demux/1 -> Alpha Lookup/1
  Cld LRBF/1 -> Mux1/4
  Cmd LRBF/1 -> Mux1/5
  Cnd LRBF/1 -> Mux1/6
  Mux1/1 -> Coeff/1
  Deltas Lower BFlap/2 -> CXd LRBF/8, Cld LRBF/8, Cmd LRBF/8, Cnd LRBF/8, CYd LRBF/8, CZd LRBF/8
  Deltas Lower BFlap/1 -> CXd LRBF/7, Cld LRBF/7, Cmd LRBF/7, Cnd LRBF/7, CYd LRBF/7, CZd LRBF/7
  Beta Lookup/2 -> Cld LRBF/6, CXd LRBF/6, Cmd LRBF/6, CYd LRBF/6, Cnd LRBF/6, CZd LRBF/6
  Beta Lookup/1 -> Cld LRBF/5, CXd LRBF/5, Cmd LRBF/5, CYd LRBF/5, Cnd LRBF/5, CZd LRBF/5
  Mach Lookup/2 -> Cnd LRBF/4, CZd LRBF/4, Cmd LRBF/4, CYd LRBF/4, CXd LRBF/4, Cld LRBF/4
  Mach Lookup/1 -> Cnd LRBF/3, CZd LRBF/3, Cmd LRBF/3, CYd LRBF/3, CXd LRBF/3, Cld LRBF/3
  Alpha Lookup/2 -> Cnd LRBF/2, CZd LRBF/2, Cmd LRBF/2, CYd LRBF/2, Cld LRBF/2, CXd LRBF/2
  Alpha Lookup/1 -> Cnd LRBF/1, CZd LRBF/1, Cmd LRBF/1, CYd LRBF/1, Cld LRBF/1, CXd LRBF/1
  albet/1 -> Demux/1
  Bus Selector1/1 -> Deltas Lower BFlap/1  "<Bflap_LoRht>"
  delta/1 -> Bus Selector1/1

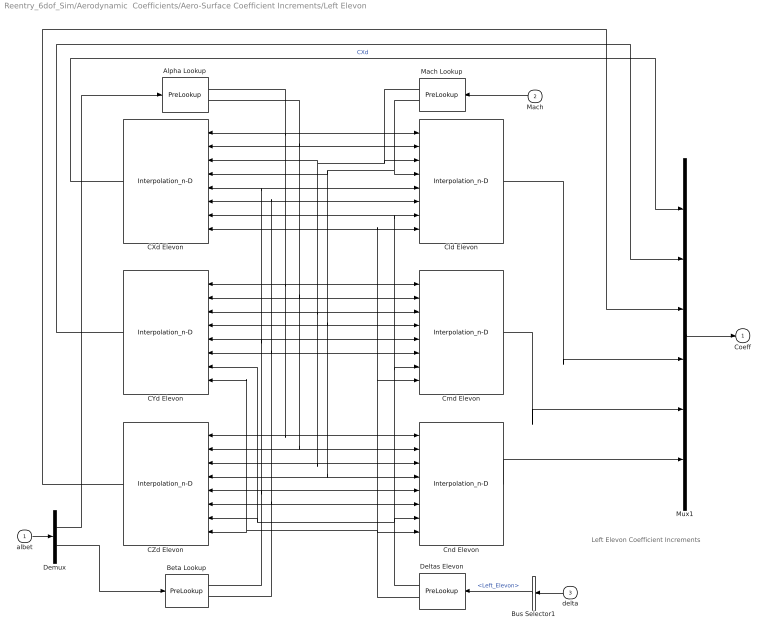
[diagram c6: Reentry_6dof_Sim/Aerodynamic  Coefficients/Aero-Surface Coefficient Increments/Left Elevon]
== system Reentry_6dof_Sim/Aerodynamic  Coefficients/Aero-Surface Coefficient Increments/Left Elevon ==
  note: Left Elevon Coefficient Increments
  albet : Inport  OutDataType=sfix(16)  OutScaling=2^0
  Mach : Inport  Port=2  OutDataType=sfix(16)  OutScaling=2^0
  delta : Inport  Port=3  OutDataType=sfix(16)  OutScaling=2^0
  Alpha Lookup : PreLookup  BreakpointsData=Alfas  BeginIndexSearchUsingPreviousIndexResult=on  ProcessOutOfRangeInput=Linear extrapolation  IndexDataType=sfix(16)  FractionDataType=sfix(16)  FractionScaling=2^0
  Beta Lookup : PreLookup  BreakpointsData=Betas  BeginIndexSearchUsingPreviousIndexResult=on  ProcessOutOfRangeInput=Linear extrapolation  IndexDataType=sfix(16)  FractionDataType=sfix(16)  FractionScaling=2^0
  Bus Selector1 : BusSelector  OutputSignals=Left_Elevon
  CXd Elevon : Interpolation_n-D  NumberOfTableDimensions=4  Table=CXd1  CheckIndexInCode=off  OutDataType=sfix(16)  OutScaling=2^0
  CYd Elevon : Interpolation_n-D  NumberOfTableDimensions=4  Table=CYd1  CheckIndexInCode=off  OutDataType=sfix(16)  OutScaling=2^0
  CZd Elevon : Interpolation_n-D  NumberOfTableDimensions=4  Table=CZd1  CheckIndexInCode=off  OutDataType=sfix(16)  OutScaling=2^0
  Cld Elevon : Interpolation_n-D  NumberOfTableDimensions=4  Table=Cld1  CheckIndexInCode=off  OutDataType=sfix(16)  OutScaling=2^0
  Cmd Elevon : Interpolation_n-D  NumberOfTableDimensions=4  Table=Cmd1  CheckIndexInCode=off  OutDataType=sfix(16)  OutScaling=2^0
  Cnd Elevon : Interpolation_n-D  NumberOfTableDimensions=4  Table=Cnd1  CheckIndexInCode=off  OutDataType=sfix(16)  OutScaling=2^0
  Deltas Elevon : PreLookup  BreakpointsData=Deltas1  BeginIndexSearchUsingPreviousIndexResult=on  ProcessOutOfRangeInput=Linear extrapolation  IndexDataType=sfix(16)  FractionDataType=sfix(16)  FractionScaling=2^0
  Demux : Demux  Outputs=2
  Mach Lookup : PreLookup  BreakpointsData=Machs  BeginIndexSearchUsingPreviousIndexResult=on  ProcessOutOfRangeInput=Linear extrapolation  IndexDataType=sfix(16)  FractionDataType=sfix(16)  FractionScaling=2^0
  Mux1 : Mux  Inputs=6
  Coeff : Outport  OutDataType=sfix(16)  OutScaling=2^0  InitialOutput=0
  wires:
  CZd Elevon/1 -> Mux1/3
  CYd Elevon/1 -> Mux1/2
  CXd Elevon/1 -> Mux1/1  "CXd"
  Demux/2 -> Beta Lookup/1
  Mach/1 -> Mach Lookup/1
  Demux/1 -> Alpha Lookup/1
  Cld Elevon/1 -> Mux1/4
  Cmd Elevon/1 -> Mux1/5
  Cnd Elevon/1 -> Mux1/6
  Mux1/1 -> Coeff/1
  Deltas Elevon/2 -> CXd Elevon/8, Cld Elevon/8, Cmd Elevon/8, Cnd Elevon/8, CYd Elevon/8, CZd Elevon/8
  Deltas Elevon/1 -> CXd Elevon/7, Cld Elevon/7, Cmd Elevon/7, Cnd Elevon/7, CYd Elevon/7, CZd Elevon/7
  Beta Lookup/2 -> Cld Elevon/6, CXd Elevon/6, Cmd Elevon/6, CYd Elevon/6, Cnd Elevon/6, CZd Elevon/6
  Beta Lookup/1 -> Cld Elevon/5, CXd Elevon/5, Cmd Elevon/5, CYd Elevon/5, Cnd Elevon/5, CZd Elevon/5
  Mach Lookup/2 -> Cnd Elevon/4, CZd Elevon/4, Cmd Elevon/4, CYd Elevon/4, CXd Elevon/4, Cld Elevon/4
  Mach Lookup/1 -> Cnd Elevon/3, CZd Elevon/3, Cmd Elevon/3, CYd Elevon/3, CXd Elevon/3, Cld Elevon/3
  Alpha Lookup/2 -> Cnd Elevon/2, CZd Elevon/2, Cmd Elevon/2, CYd Elevon/2, Cld Elevon/2, CXd Elevon/2
  Alpha Lookup/1 -> Cnd Elevon/1, CZd Elevon/1, Cmd Elevon/1, CYd Elevon/1, Cld Elevon/1, CXd Elevon/1
  albet/1 -> Demux/1
  Bus Selector1/1 -> Deltas Elevon/1  "<Left_Elevon>"
  delta/1 -> Bus Selector1/1

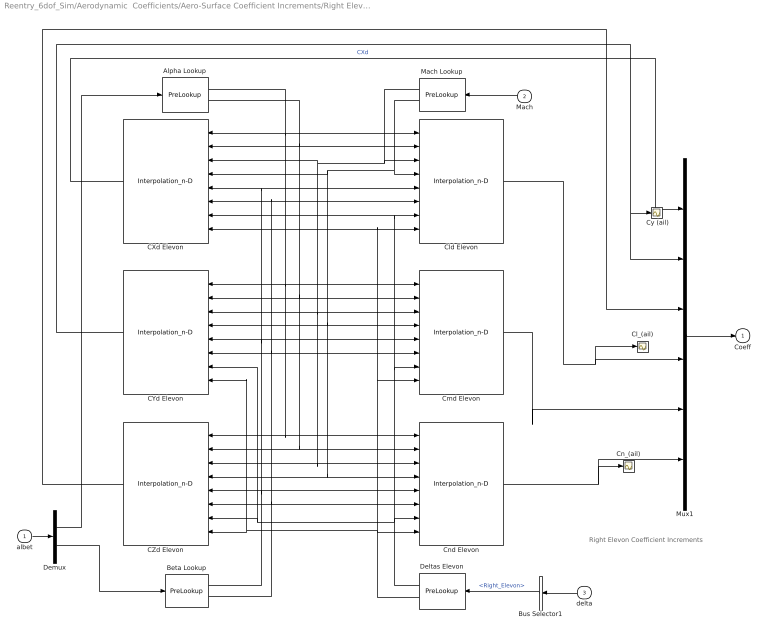
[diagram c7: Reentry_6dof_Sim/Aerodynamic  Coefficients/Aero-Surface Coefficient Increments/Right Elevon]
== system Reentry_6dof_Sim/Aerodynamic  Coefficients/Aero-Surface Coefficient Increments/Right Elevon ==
  note: Right Elevon Coefficient Increments
  albet : Inport  OutDataType=sfix(16)  OutScaling=2^0
  Mach : Inport  Port=2  OutDataType=sfix(16)  OutScaling=2^0
  delta : Inport  Port=3  OutDataType=sfix(16)  OutScaling=2^0
  " Cy (ail)" : Scope
  Alpha Lookup : PreLookup  BreakpointsData=Alfas  BeginIndexSearchUsingPreviousIndexResult=on  ProcessOutOfRangeInput=Linear extrapolation  IndexDataType=sfix(16)  FractionDataType=sfix(16)  FractionScaling=2^0
  Beta Lookup : PreLookup  BreakpointsData=Betas  BeginIndexSearchUsingPreviousIndexResult=on  ProcessOutOfRangeInput=Linear extrapolation  IndexDataType=sfix(16)  FractionDataType=sfix(16)  FractionScaling=2^0
  Bus Selector1 : BusSelector  OutputSignals=Right_Elevon
  CXd Elevon : Interpolation_n-D  NumberOfTableDimensions=4  Table=CXd2  CheckIndexInCode=off  OutDataType=sfix(16)  OutScaling=2^0
  CYd Elevon : Interpolation_n-D  NumberOfTableDimensions=4  Table=CYd2  CheckIndexInCode=off  OutDataType=sfix(16)  OutScaling=2^0
  CZd Elevon : Interpolation_n-D  NumberOfTableDimensions=4  Table=CZd2  CheckIndexInCode=off  OutDataType=sfix(16)  OutScaling=2^0
  Cl_(ail) : Scope
  Cld Elevon : Interpolation_n-D  NumberOfTableDimensions=4  Table=Cld2  CheckIndexInCode=off  OutDataType=sfix(16)  OutScaling=2^0
  Cmd Elevon : Interpolation_n-D  NumberOfTableDimensions=4  Table=Cmd2  CheckIndexInCode=off  OutDataType=sfix(16)  OutScaling=2^0
  Cn_(ail) : Scope
  Cnd Elevon : Interpolation_n-D  NumberOfTableDimensions=4  Table=Cnd2  CheckIndexInCode=off  OutDataType=sfix(16)  OutScaling=2^0
  Deltas Elevon : PreLookup  BreakpointsData=Deltas2  BeginIndexSearchUsingPreviousIndexResult=on  ProcessOutOfRangeInput=Linear extrapolation  IndexDataType=sfix(16)  FractionDataType=sfix(16)  FractionScaling=2^0
  Demux : Demux  Outputs=2
  Mach Lookup : PreLookup  BreakpointsData=Machs  BeginIndexSearchUsingPreviousIndexResult=on  ProcessOutOfRangeInput=Linear extrapolation  IndexDataType=sfix(16)  FractionDataType=sfix(16)  FractionScaling=2^0
  Mux1 : Mux  Inputs=6
  Coeff : Outport  OutDataType=sfix(16)  OutScaling=2^0  InitialOutput=0
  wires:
  CZd Elevon/1 -> Mux1/3
  CYd Elevon/1 -> Mux1/2, " Cy (ail)"/1
  CXd Elevon/1 -> Mux1/1  "CXd"
  delta/1 -> Bus Selector1/1
  Demux/2 -> Beta Lookup/1
  Mach/1 -> Mach Lookup/1
  Demux/1 -> Alpha Lookup/1
  Cld Elevon/1 -> Mux1/4, Cl_(ail)/1
  Cmd Elevon/1 -> Mux1/5
  Cnd Elevon/1 -> Mux1/6, Cn_(ail)/1
  Mux1/1 -> Coeff/1
  Deltas Elevon/2 -> CXd Elevon/8, Cld Elevon/8, Cmd Elevon/8, Cnd Elevon/8, CYd Elevon/8, CZd Elevon/8
  Deltas Elevon/1 -> CXd Elevon/7, Cld Elevon/7, Cmd Elevon/7, Cnd Elevon/7, CYd Elevon/7, CZd Elevon/7
  Beta Lookup/2 -> Cld Elevon/6, CXd Elevon/6, Cmd Elevon/6, CYd Elevon/6, Cnd Elevon/6, CZd Elevon/6
  Beta Lookup/1 -> Cld Elevon/5, CXd Elevon/5, Cmd Elevon/5, CYd Elevon/5, Cnd Elevon/5, CZd Elevon/5
  Mach Lookup/2 -> Cnd Elevon/4, CZd Elevon/4, Cmd Elevon/4, CYd Elevon/4, CXd Elevon/4, Cld Elevon/4
  Mach Lookup/1 -> Cnd Elevon/3, CZd Elevon/3, Cmd Elevon/3, CYd Elevon/3, CXd Elevon/3, Cld Elevon/3
  Alpha Lookup/2 -> Cnd Elevon/2, CZd Elevon/2, Cmd Elevon/2, CYd Elevon/2, Cld Elevon/2, CXd Elevon/2
  Alpha Lookup/1 -> Cnd Elevon/1, CZd Elevon/1, Cmd Elevon/1, CYd Elevon/1, Cld Elevon/1, CXd Elevon/1
  albet/1 -> Demux/1
  Bus Selector1/1 -> Deltas Elevon/1  "<Right_Elevon>"

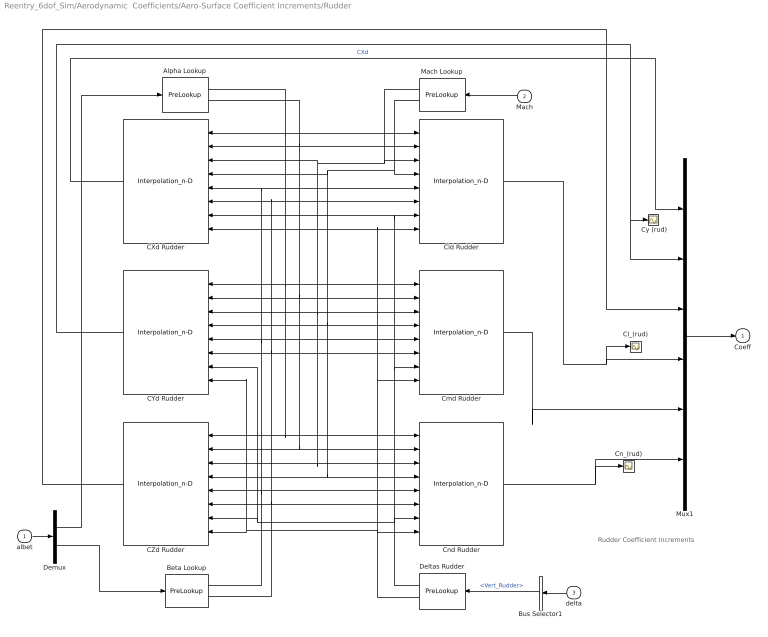
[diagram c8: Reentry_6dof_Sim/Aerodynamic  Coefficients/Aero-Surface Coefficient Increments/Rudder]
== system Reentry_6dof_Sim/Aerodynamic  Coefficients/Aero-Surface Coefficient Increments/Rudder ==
  note: Rudder Coefficient Increments
  albet : Inport  OutDataType=sfix(16)  OutScaling=2^0
  Mach : Inport  Port=2  OutDataType=sfix(16)  OutScaling=2^0
  delta : Inport  Port=3  OutDataType=sfix(16)  OutScaling=2^0
  " Cy (rud)" : Scope
  Alpha Lookup : PreLookup  BreakpointsData=Alfas  BeginIndexSearchUsingPreviousIndexResult=on  ProcessOutOfRangeInput=Linear extrapolation  IndexDataType=sfix(16)  FractionDataType=sfix(16)  FractionScaling=2^0
  Beta Lookup : PreLookup  BreakpointsData=Betas  BeginIndexSearchUsingPreviousIndexResult=on  ProcessOutOfRangeInput=Linear extrapolation  IndexDataType=sfix(16)  FractionDataType=sfix(16)  FractionScaling=2^0
  Bus Selector1 : BusSelector  OutputSignals=Vert_Rudder
  CXd Rudder : Interpolation_n-D  NumberOfTableDimensions=4  Table=CXd3  CheckIndexInCode=off  OutDataType=sfix(16)  OutScaling=2^0
  CYd Rudder : Interpolation_n-D  NumberOfTableDimensions=4  Table=CYd3  CheckIndexInCode=off  OutDataType=sfix(16)  OutScaling=2^0
  CZd Rudder : Interpolation_n-D  NumberOfTableDimensions=4  Table=CZd3  CheckIndexInCode=off  OutDataType=sfix(16)  OutScaling=2^0
  Cl_(rud) : Scope
  Cld Rudder : Interpolation_n-D  NumberOfTableDimensions=4  Table=Cld3  CheckIndexInCode=off  OutDataType=sfix(16)  OutScaling=2^0
  Cmd Rudder : Interpolation_n-D  NumberOfTableDimensions=4  Table=Cmd3  CheckIndexInCode=off  OutDataType=sfix(16)  OutScaling=2^0
  Cn_(rud) : Scope
  Cnd Rudder : Interpolation_n-D  NumberOfTableDimensions=4  Table=Cnd3  CheckIndexInCode=off  OutDataType=sfix(16)  OutScaling=2^0
  Deltas Rudder : PreLookup  BreakpointsData=Deltas3  BeginIndexSearchUsingPreviousIndexResult=on  ProcessOutOfRangeInput=Linear extrapolation  IndexDataType=sfix(16)  FractionDataType=sfix(16)  FractionScaling=2^0
  Demux : Demux  Outputs=2
  Mach Lookup : PreLookup  BreakpointsData=Machs  BeginIndexSearchUsingPreviousIndexResult=on  ProcessOutOfRangeInput=Linear extrapolation  IndexDataType=sfix(16)  FractionDataType=sfix(16)  FractionScaling=2^0
  Mux1 : Mux  Inputs=6
  Coeff : Outport  OutDataType=sfix(16)  OutScaling=2^0  InitialOutput=0
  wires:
  CZd Rudder/1 -> Mux1/3
  CYd Rudder/1 -> Mux1/2, " Cy (rud)"/1
  CXd Rudder/1 -> Mux1/1  "CXd"
  delta/1 -> Bus Selector1/1
  Demux/2 -> Beta Lookup/1
  Mach/1 -> Mach Lookup/1
  Demux/1 -> Alpha Lookup/1
  Cld Rudder/1 -> Mux1/4, Cl_(rud)/1
  Cmd Rudder/1 -> Mux1/5
  Cnd Rudder/1 -> Mux1/6, Cn_(rud)/1
  Mux1/1 -> Coeff/1
  Deltas Rudder/2 -> CXd Rudder/8, Cld Rudder/8, Cmd Rudder/8, Cnd Rudder/8, CYd Rudder/8, CZd Rudder/8
  Deltas Rudder/1 -> CXd Rudder/7, Cld Rudder/7, Cmd Rudder/7, Cnd Rudder/7, CYd Rudder/7, CZd Rudder/7
  Beta Lookup/2 -> Cld Rudder/6, CXd Rudder/6, Cmd Rudder/6, CYd Rudder/6, Cnd Rudder/6, CZd Rudder/6
  Beta Lookup/1 -> Cld Rudder/5, CXd Rudder/5, Cmd Rudder/5, CYd Rudder/5, Cnd Rudder/5, CZd Rudder/5
  Mach Lookup/2 -> Cnd Rudder/4, CZd Rudder/4, Cmd Rudder/4, CYd Rudder/4, CXd Rudder/4, Cld Rudder/4
  Mach Lookup/1 -> Cnd Rudder/3, CZd Rudder/3, Cmd Rudder/3, CYd Rudder/3, CXd Rudder/3, Cld Rudder/3
  Alpha Lookup/2 -> Cnd Rudder/2, CZd Rudder/2, Cmd Rudder/2, CYd Rudder/2, Cld Rudder/2, CXd Rudder/2
  Alpha Lookup/1 -> Cnd Rudder/1, CZd Rudder/1, Cmd Rudder/1, CYd Rudder/1, Cld Rudder/1, CXd Rudder/1
  albet/1 -> Demux/1
  Bus Selector1/1 -> Deltas Rudder/1  "<Vert_Rudder>"

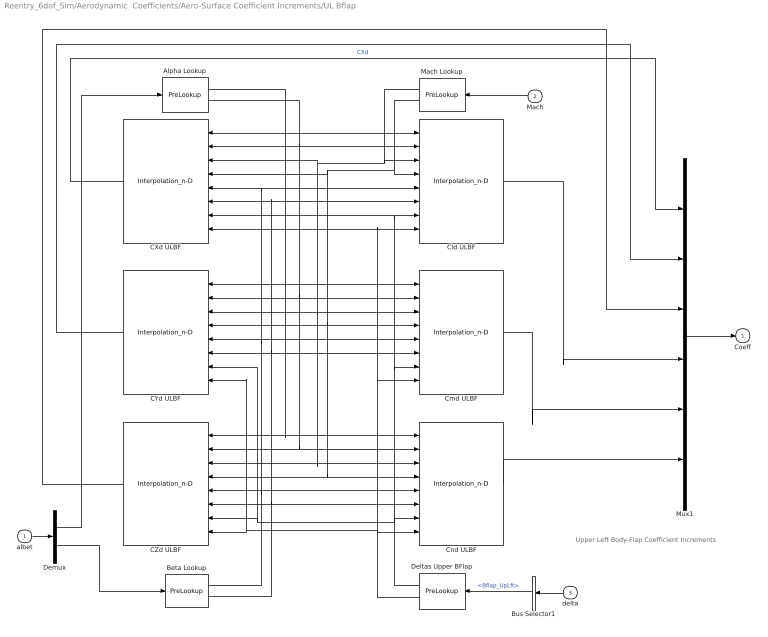
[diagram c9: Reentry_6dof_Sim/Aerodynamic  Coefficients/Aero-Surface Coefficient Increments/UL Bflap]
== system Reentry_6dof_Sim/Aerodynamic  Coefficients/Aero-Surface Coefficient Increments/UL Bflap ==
  note: Upper Left Body-Flap Coefficient Increments
  albet : Inport  OutDataType=sfix(16)  OutScaling=2^0
  Mach : Inport  Port=2  OutDataType=sfix(16)  OutScaling=2^0
  delta : Inport  Port=3  OutDataType=sfix(16)  OutScaling=2^0
  Alpha Lookup : PreLookup  BreakpointsData=Alfas  BeginIndexSearchUsingPreviousIndexResult=on  ProcessOutOfRangeInput=Linear extrapolation  IndexDataType=sfix(16)  FractionDataType=sfix(16)  FractionScaling=2^0
  Beta Lookup : PreLookup  BreakpointsData=Betas  BeginIndexSearchUsingPreviousIndexResult=on  ProcessOutOfRangeInput=Linear extrapolation  IndexDataType=sfix(16)  FractionDataType=sfix(16)  FractionScaling=2^0
  Bus Selector1 : BusSelector  OutputSignals=Bflap_UpLft
  CXd ULBF : Interpolation_n-D  NumberOfTableDimensions=4  Table=CXd4  CheckIndexInCode=off  OutDataType=sfix(16)  OutScaling=2^0
  CYd ULBF : Interpolation_n-D  NumberOfTableDimensions=4  Table=CYd4  CheckIndexInCode=off  OutDataType=sfix(16)  OutScaling=2^0
  CZd ULBF : Interpolation_n-D  NumberOfTableDimensions=4  Table=CZd4  CheckIndexInCode=off  OutDataType=sfix(16)  OutScaling=2^0
  Cld ULBF : Interpolation_n-D  NumberOfTableDimensions=4  Table=Cld4  CheckIndexInCode=off  OutDataType=sfix(16)  OutScaling=2^0
  Cmd ULBF : Interpolation_n-D  NumberOfTableDimensions=4  Table=Cmd4  CheckIndexInCode=off  OutDataType=sfix(16)  OutScaling=2^0
  Cnd ULBF : Interpolation_n-D  NumberOfTableDimensions=4  Table=Cnd4  CheckIndexInCode=off  OutDataType=sfix(16)  OutScaling=2^0
  Deltas Upper BFlap : PreLookup  BreakpointsData=Deltas4  BeginIndexSearchUsingPreviousIndexResult=on  ProcessOutOfRangeInput=Linear extrapolation  IndexDataType=sfix(16)  FractionDataType=sfix(16)  FractionScaling=2^0
  Demux : Demux  Outputs=2
  Mach Lookup : PreLookup  BreakpointsData=Machs  BeginIndexSearchUsingPreviousIndexResult=on  ProcessOutOfRangeInput=Linear extrapolation  IndexDataType=sfix(16)  FractionDataType=sfix(16)  FractionScaling=2^0
  Mux1 : Mux  Inputs=6
  Coeff : Outport  OutDataType=sfix(16)  OutScaling=2^0  InitialOutput=0
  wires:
  CZd ULBF/1 -> Mux1/3
  CYd ULBF/1 -> Mux1/2
  CXd ULBF/1 -> Mux1/1  "CXd"
  Demux/2 -> Beta Lookup/1
  Mach/1 -> Mach Lookup/1
  Demux/1 -> Alpha Lookup/1
  Cld ULBF/1 -> Mux1/4
  Cmd ULBF/1 -> Mux1/5
  Cnd ULBF/1 -> Mux1/6
  Mux1/1 -> Coeff/1
  Deltas Upper BFlap/2 -> CXd ULBF/8, Cld ULBF/8, Cmd ULBF/8, Cnd ULBF/8, CYd ULBF/8, CZd ULBF/8
  Deltas Upper BFlap/1 -> CXd ULBF/7, Cld ULBF/7, Cmd ULBF/7, Cnd ULBF/7, CYd ULBF/7, CZd ULBF/7
  Beta Lookup/2 -> Cld ULBF/6, CXd ULBF/6, Cmd ULBF/6, CYd ULBF/6, Cnd ULBF/6, CZd ULBF/6
  Beta Lookup/1 -> Cld ULBF/5, CXd ULBF/5, Cmd ULBF/5, CYd ULBF/5, Cnd ULBF/5, CZd ULBF/5
  Mach Lookup/2 -> Cnd ULBF/4, CZd ULBF/4, Cmd ULBF/4, CYd ULBF/4, CXd ULBF/4, Cld ULBF/4
  Mach Lookup/1 -> Cnd ULBF/3, CZd ULBF/3, Cmd ULBF/3, CYd ULBF/3, CXd ULBF/3, Cld ULBF/3
  Alpha Lookup/2 -> Cnd ULBF/2, CZd ULBF/2, Cmd ULBF/2, CYd ULBF/2, Cld ULBF/2, CXd ULBF/2
  Alpha Lookup/1 -> Cnd ULBF/1, CZd ULBF/1, Cmd ULBF/1, CYd ULBF/1, Cld ULBF/1, CXd ULBF/1
  albet/1 -> Demux/1
  Bus Selector1/1 -> Deltas Upper BFlap/1  "<Bflap_UpLft>"
  delta/1 -> Bus Selector1/1

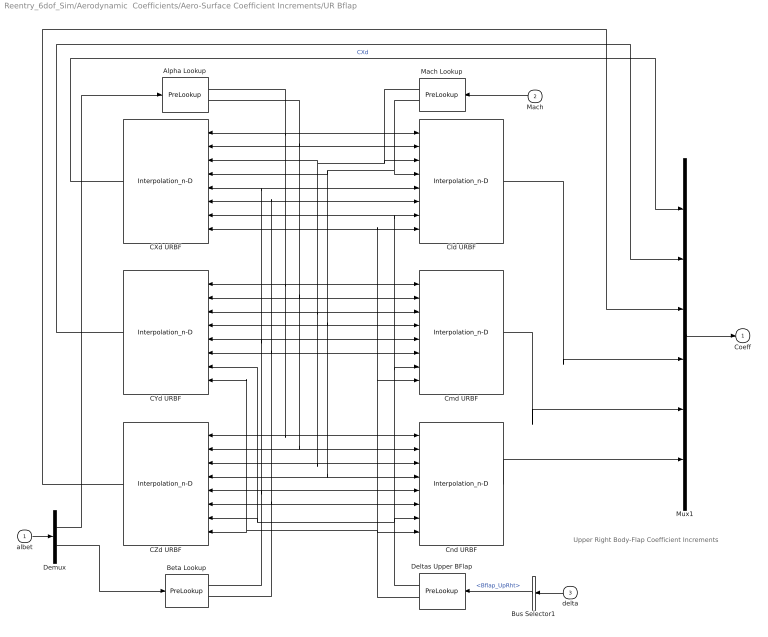
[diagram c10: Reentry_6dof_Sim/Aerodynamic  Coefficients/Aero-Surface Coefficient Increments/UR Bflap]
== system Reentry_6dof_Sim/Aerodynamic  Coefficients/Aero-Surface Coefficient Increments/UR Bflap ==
  note: Upper Right Body-Flap Coefficient Increments
  albet : Inport  OutDataType=sfix(16)  OutScaling=2^0
  Mach : Inport  Port=2  OutDataType=sfix(16)  OutScaling=2^0
  delta : Inport  Port=3  OutDataType=sfix(16)  OutScaling=2^0
  Alpha Lookup : PreLookup  BreakpointsData=Alfas  BeginIndexSearchUsingPreviousIndexResult=on  ProcessOutOfRangeInput=Linear extrapolation  IndexDataType=sfix(16)  FractionDataType=sfix(16)  FractionScaling=2^0
  Beta Lookup : PreLookup  BreakpointsData=Betas  BeginIndexSearchUsingPreviousIndexResult=on  ProcessOutOfRangeInput=Linear extrapolation  IndexDataType=sfix(16)  FractionDataType=sfix(16)  FractionScaling=2^0
  Bus Selector1 : BusSelector  OutputSignals=Bflap_UpRht
  CXd URBF : Interpolation_n-D  NumberOfTableDimensions=4  Table=CXd5  CheckIndexInCode=off  OutDataType=sfix(16)  OutScaling=2^0
  CYd URBF : Interpolation_n-D  NumberOfTableDimensions=4  Table=CYd5  CheckIndexInCode=off  OutDataType=sfix(16)  OutScaling=2^0
  CZd URBF : Interpolation_n-D  NumberOfTableDimensions=4  Table=CZd5  CheckIndexInCode=off  OutDataType=sfix(16)  OutScaling=2^0
  Cld URBF : Interpolation_n-D  NumberOfTableDimensions=4  Table=Cld5  CheckIndexInCode=off  OutDataType=sfix(16)  OutScaling=2^0
  Cmd URBF : Interpolation_n-D  NumberOfTableDimensions=4  Table=Cmd5  CheckIndexInCode=off  OutDataType=sfix(16)  OutScaling=2^0
  Cnd URBF : Interpolation_n-D  NumberOfTableDimensions=4  Table=Cnd5  CheckIndexInCode=off  OutDataType=sfix(16)  OutScaling=2^0
  Deltas Upper BFlap : PreLookup  BreakpointsData=Deltas5  BeginIndexSearchUsingPreviousIndexResult=on  ProcessOutOfRangeInput=Linear extrapolation  IndexDataType=sfix(16)  FractionDataType=sfix(16)  FractionScaling=2^0
  Demux : Demux  Outputs=2
  Mach Lookup : PreLookup  BreakpointsData=Machs  BeginIndexSearchUsingPreviousIndexResult=on  ProcessOutOfRangeInput=Linear extrapolation  IndexDataType=sfix(16)  FractionDataType=sfix(16)  FractionScaling=2^0
  Mux1 : Mux  Inputs=6
  Coeff : Outport  OutDataType=sfix(16)  OutScaling=2^0  InitialOutput=0
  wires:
  CZd URBF/1 -> Mux1/3
  CYd URBF/1 -> Mux1/2
  CXd URBF/1 -> Mux1/1  "CXd"
  Demux/2 -> Beta Lookup/1
  Mach/1 -> Mach Lookup/1
  Demux/1 -> Alpha Lookup/1
  Cld URBF/1 -> Mux1/4
  Cmd URBF/1 -> Mux1/5
  Cnd URBF/1 -> Mux1/6
  Mux1/1 -> Coeff/1
  Deltas Upper BFlap/2 -> CXd URBF/8, Cld URBF/8, Cmd URBF/8, Cnd URBF/8, CYd URBF/8, CZd URBF/8
  Deltas Upper BFlap/1 -> CXd URBF/7, Cld URBF/7, Cmd URBF/7, Cnd URBF/7, CYd URBF/7, CZd URBF/7
  Beta Lookup/2 -> Cld URBF/6, CXd URBF/6, Cmd URBF/6, CYd URBF/6, Cnd URBF/6, CZd URBF/6
  Beta Lookup/1 -> Cld URBF/5, CXd URBF/5, Cmd URBF/5, CYd URBF/5, Cnd URBF/5, CZd URBF/5
  Mach Lookup/2 -> Cnd URBF/4, CZd URBF/4, Cmd URBF/4, CYd URBF/4, CXd URBF/4, Cld URBF/4
  Mach Lookup/1 -> Cnd URBF/3, CZd URBF/3, Cmd URBF/3, CYd URBF/3, CXd URBF/3, Cld URBF/3
  Alpha Lookup/2 -> Cnd URBF/2, CZd URBF/2, Cmd URBF/2, CYd URBF/2, Cld URBF/2, CXd URBF/2
  Alpha Lookup/1 -> Cnd URBF/1, CZd URBF/1, Cmd URBF/1, CYd URBF/1, Cld URBF/1, CXd URBF/1
  albet/1 -> Demux/1
  Bus Selector1/1 -> Deltas Upper BFlap/1  "<Bflap_UpRht>"
  delta/1 -> Bus Selector1/1

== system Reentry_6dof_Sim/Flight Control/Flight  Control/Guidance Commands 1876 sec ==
  Demux : Demux  Tag=STV Demux  Outputs=2
  FromWs : FromWorkspace  Tag=STV FromWs  VariableName=tuvar  SampleTime=0  SigBuilderData=DataTag0  VnvData=DataTag1
  Alpha_cmd : Outport  Tag=STV Outport
  Gamma_cmd : Outport  Tag=STV Outport  Port=2
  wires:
  FromWs/1 -> Demux/1
  Demux/1 -> Alpha_cmd/1
  Demux/2 -> Gamma_cmd/1

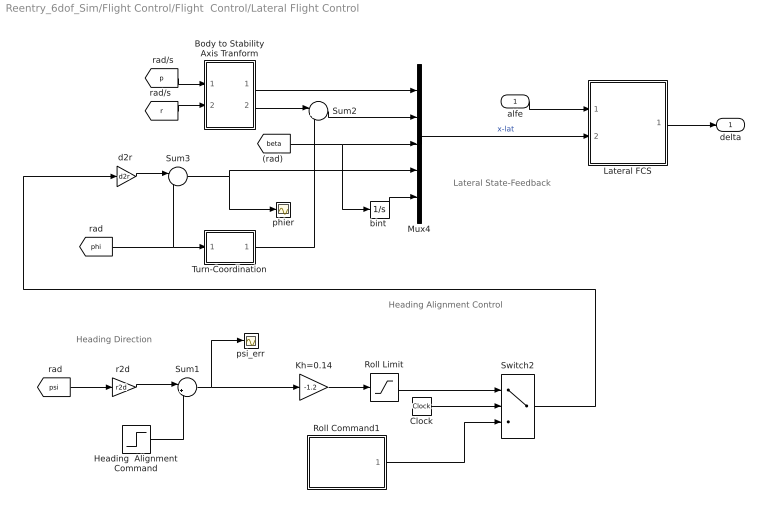
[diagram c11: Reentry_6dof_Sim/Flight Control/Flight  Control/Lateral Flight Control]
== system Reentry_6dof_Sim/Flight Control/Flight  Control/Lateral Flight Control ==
  note: Lateral State-Feedback
  note: Heading Alignment Control
  note: Heading Direction
  alfe : Inport
  Body to Stability Axis Tranform : Subsystem
  Clock : Clock
  Heading  Alignment Command : Step  Time=1560  Before=1.8  After=-70  SampleTime=0
  Kh=0.14 : Gain  Gain=-1.2  ParameterDataType=sfix(16)  ParameterScaling=2^0  OutDataType=sfix(16)  OutScaling=2^0
  Lateral FCS : Subsystem
  Mux4 : Mux  Inputs=5
  Roll Limit : Saturate  UpperLimit=40  LowerLimit=-40  OutDataType=fixdt(1, 16)  OutScaling=2^0
  Roll Command1 : Subsystem  Tag=STV Subsys  LoadFcn=sigbuilder_block('load');  StartFcn=sigbuilder_block('start');  StopFcn=sigbuilder_block('stop');  ClipboardFcn=sigbuilder_block('clipboard');
  Sum1 : Sum  Inputs=|+-  OutDataType=sfix(16)  OutScaling=2^0
  Sum2 : Sum  Inputs=|++  OutDataType=fixdt(1, 16)  OutScaling=2^0
  Sum3 : Sum  Inputs=|-+  OutDataType=fixdt(1, 16)  OutScaling=2^0
  Switch2 : Switch  Threshold=1400  OutDataType=fixdt(1, 16)  OutScaling=2^0
  Turn-Coordination : Subsystem
  "bint " : Integrator
  "d2r " : Gain  Gain=d2r  ParameterDataType=fixdt(1, 16)  ParameterScaling=2^0  OutDataType=fixdt(1, 16)  OutScaling=2^0
  phier : Scope
  psi_err : Scope
  "r2d " : Gain  Gain=r2d  ParameterDataType=sfix(16)  ParameterScaling=2^0  OutDataType=sfix(16)  OutScaling=2^0
  delta : Outport
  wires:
  Sum3/1 -> Mux4/4, phier/1
  "d2r "/1 -> Sum3/1
  [p] -> Body to Stability Axis Tranform/1(p_b)
  [r] -> Body to Stability Axis Tranform/2(r_b)
  Body to Stability Axis Tranform/1(p_s) -> Mux4/1
  [beta] -> Mux4/3, "bint "/1
  Body to Stability Axis Tranform/2(r_s) -> Sum2/1
  Sum2/1 -> Mux4/2
  Mux4/1 -> Lateral FCS/2(xlat)  "x-lat"
  alfe/1 -> Lateral FCS/1(ae)
  Lateral FCS/1(delta) -> delta/1
  "bint "/1 -> Mux4/5
  Turn-Coordination/1(Rff) -> Sum2/2
  [phi] -> Sum3/2, Turn-Coordination/1(phi)
  "r2d "/1 -> Sum1/1
  [psi] -> "r2d "/1
  Kh=0.14/1 -> Roll Limit/1
  Roll Command1/1(Phi_cmd) -> Switch2/3
  Clock/1 -> Switch2/2
  Sum1/1 -> psi_err/1, Kh=0.14/1
  Heading  Alignment Command/1 -> Sum1/2
  Roll Limit/1 -> Switch2/1
  Switch2/1 -> "d2r "/1

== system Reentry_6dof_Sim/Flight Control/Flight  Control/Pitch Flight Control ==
  note: Pitch State-Feedback
  gamer : Inport
  alfer : Inport  Port=2
  " d2r" : Gain  Gain=d2r  ParameterDataType=fixdt(1, 16)  ParameterScaling=2^0  OutDataType=fixdt(1, 16)  OutScaling=2^0
  Gains Interpolator : Subsystem
  Mux2 : Mux  Inputs=7
  NZ-filtr : TransferFcn  Numerator=[20]  Denominator=[1 20]
  Nz Command : Subsystem  Tag=STV Subsys  LoadFcn=sigbuilder_block('load');  StartFcn=sigbuilder_block('start');  StopFcn=sigbuilder_block('stop');  ClipboardFcn=sigbuilder_block('clipboard');
  Sum4 : Sum  Inputs=|++  OutDataType=fixdt(1, 16)  OutScaling=2^0
  alfin : Integrator
  intgr : Subsystem
  intgr1 : Subsystem
  r2d : Gain  Gain=r2d  ParameterDataType=fixdt(1, 16)  ParameterScaling=2^0  OutDataType=fixdt(1, 16)  OutScaling=2^0
  delta : Outport
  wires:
  [q] -> Mux2/3  "q"
  alfer/1 -> alfin/1, r2d/1, Mux2/4  "alfer"
  r2d/1 -> Gains Interpolator/2(alferr)
  intgr/1(gi) -> Mux2/1  "gami"
  alfin/1 -> Mux2/5  "alfin"
  " d2r"/1 -> intgr/1(ge), Mux2/2  "gamer"
  Mux2/1 -> Gains Interpolator/1(xq)  "x-ptch"
  gamer/1 -> " d2r"/1
  Gains Interpolator/1(Deltas) -> delta/1
  Nz Command/1(Nz_cmd) -> Sum4/2
  [Nz] -> Sum4/1
  intgr1/1(nzi) -> Mux2/7
  NZ-filtr/1 -> Mux2/6, intgr1/1(nze)
  Sum4/1 -> NZ-filtr/1
